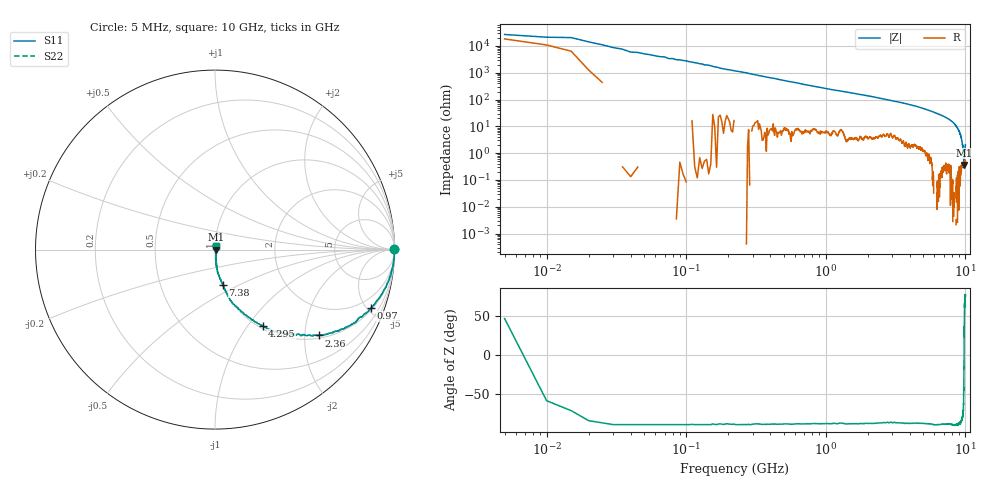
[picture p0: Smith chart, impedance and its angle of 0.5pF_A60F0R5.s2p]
! Amotech Co.,Ltd.
! http://www.amotech.co.kr/
! Part Number: A60F0R5
! These Parameters are Measured in Series Mode Connection
! Operation Temp=25[degC], DC Bias Voltage=0[V]
! Freq. Start=5[MHz] Stop=10[GHz], 2000[Steps]
! Date: Monday, July 20, 2020, 03:11:03
# GHZ S RI R 50.000000
!Freq.(Hz) S11(Real) S11(Imag) S21(Real) S21(Imag) S12(Real) S12(Imag) S22(Real) S22(Imag)
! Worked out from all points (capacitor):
!   2000 points, 5 MHz to 10 GHz, reference 50 ohm
!   read as one part in series: C = 584 fF near 55 MHz
!   lowest |Z| = 364 mohm at 9.78 GHz (marker M1)
!   series resonance near 9.78 GHz, so ESL is about 450 pH
!   S11 on the Smith chart (normalised r, x): 5 MHz: open; 970 MHz: 1.12, -5.32; 2.36 GHz: 1.08, -2.35; 4.295 GHz: 1.04, -1.18; 7.38 GHz: 1.01, -0.41; 10 GHz: 1.01, +0.04
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0.005  0.9975 0.00269  0.00252 -0.00269  0.00252 -0.00269  0.9975 0.00269
0.09  0.9989 -0.0327  0.00108 0.0327  0.00108 0.0327  0.9989 -0.0327
0.155  0.9959 -0.0566  0.00412 0.0566  0.00412 0.0566  0.9959 -0.0566
0.235  0.9924 -0.087  0.00763 0.087  0.00763 0.087  0.9924 -0.087
0.525  0.9577 -0.1931  0.0423 0.1931  0.0423 0.1931  0.9577 -0.1931
0.97  0.8708 -0.3244  0.1292 0.3244  0.1292 0.3244  0.8708 -0.3244
1.675  0.7241 -0.437  0.2759 0.437  0.2759 0.437  0.7241 -0.437
2.36  0.5768 -0.478  0.4232 0.478  0.4232 0.478  0.5768 -0.478
3.34  0.3947 -0.4699  0.6053 0.4699  0.6053 0.4699  0.3947 -0.4699
4.295  0.265 -0.4243  0.735 0.4243  0.735 0.4243  0.265 -0.4243
5.005  0.1829 -0.3744  0.8171 0.3744  0.8171 0.3744  0.1829 -0.3744
6.67  0.0667 -0.2467  0.9333 0.2467  0.9333 0.2467  0.0667 -0.2467
7.38  0.043 -0.1947  0.957 0.1947  0.957 0.1947  0.043 -0.1947
8.335  0.0132 -0.1221  0.9868 0.1221  0.9868 0.1221  0.0132 -0.1221
8.89  0.00776 -0.0762  0.9922 0.0762  0.9922 0.0762  0.00776 -0.0762
9.28  0.00413 -0.0423  0.9959 0.0423  0.9959 0.0423  0.00413 -0.0423
9.565  0.00375 -0.0176  0.9962 0.0176  0.9962 0.0176  0.00375 -0.0176
9.74  0.00412 -0.00422  0.9959 0.00422  0.9959 0.00422  0.00412 -0.00422
9.78  0.00362 0.000132  0.9964 -0.000132  0.9964 -0.000132  0.00362 0.000132
9.82  0.00437 0.00345  0.9956 -0.00345  0.9956 -0.00345  0.00437 0.00345
9.925  0.00502 0.0137  0.995 -0.0137  0.995 -0.0137  0.00502 0.0137
10  0.0054 0.0197  0.9946 -0.0197  0.9946 -0.0197  0.0054 0.0197
